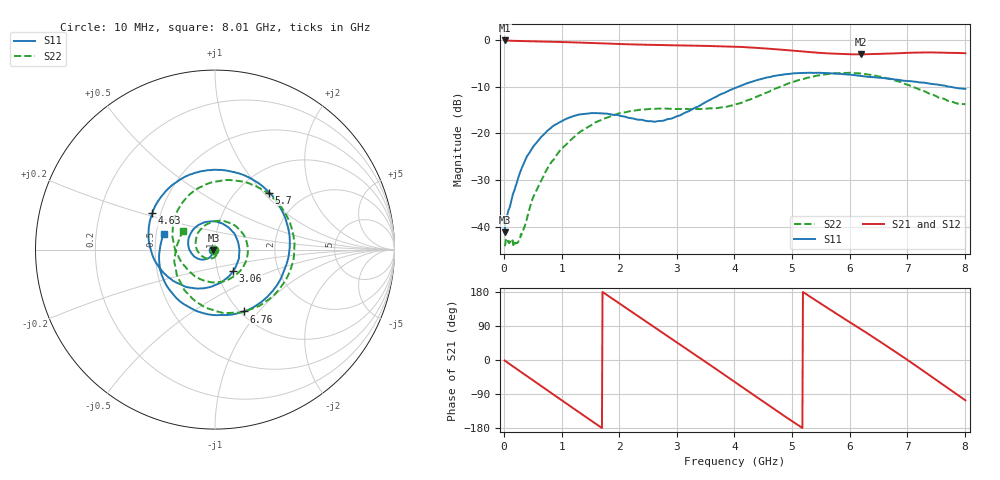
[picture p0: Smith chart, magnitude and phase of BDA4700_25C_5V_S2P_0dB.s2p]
!Agilent Technologies,E5071B,MY42404982,A.09.10
!Date: Mon Oct 20 13:25:59 2025
!Data & Calibration Information:
!Freq	S11:SOLT2(ON)	S21:SOLT2(ON)	S12:SOLT2(ON)	S22:SOLT2(ON)
# Hz S RI R 50
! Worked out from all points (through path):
!   801 points, 10 MHz to 8.01 GHz, reference 50 ohm
!   highest |S21| = -0.12 dB at 10 MHz (marker M1); lowest = -3.1 dB at 6.19 GHz (marker M2)
!   group delay of S21, straight-line fit = 285 ps
!   lowest |S11| = -41.1 dB at 10 MHz (marker M3), VSWR 1.02, Z = 49.2 - j0.259 ohm
!   |S11| at or under -10 dB: start of sweep to 4.065 GHz; 7.731 GHz to end of sweep
!   |S22| runs from -44.1 to -7.0 dB; largest |S21 - S12| = 0.0073
!   S11 on the Smith chart (normalised r, x): 10 MHz: 0.98, -0.01; 3.06 GHz: 1.18, -0.29; 4.63 GHz: 0.45, +0.22; 5.7 GHz: 1.37, +1.08; 6.76 GHz: 1.04, -0.84; 8.01 GHz: 0.55, +0.10
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1e7  -0.00836 -0.00263  0.9858 -0.0211  0.9859 -0.0221  -0.00624 -0.00044
2.6e8  -0.0186 -0.0303  0.859 -0.4568  0.8594 -0.457  0.00486 0.00556
7.2e8  -0.0874 -0.053  0.2215 -0.9322  0.2211 -0.9327  0.00204 -0.0389
1.02e9  -0.1369 -0.0116  -0.2964 -0.9004  -0.297 -0.9006  -0.0519 -0.0479
1.35e9  -0.144 0.0705  -0.7449 -0.5637  -0.7455 -0.5638  -0.1056 0.0151
1.92e9  -0.0155 0.1577  -0.8401 0.3442  -0.8409 0.3448  0.000695 0.1584
2.32e9  0.0934 0.1049  -0.3984 0.7978  -0.3985 0.7981  0.1469 0.1003
2.68e9  0.1358 0.00145  0.1593 0.8677  0.1596 0.8675  0.1779 -0.0486
3.06e9  0.0992 -0.1214  0.6655 0.5653  0.6626 0.5681  0.077 -0.1658
3.52e9  -0.0496 -0.2131  0.8552 -0.1075  0.8557 -0.109  -0.0892 -0.161
4.01e9  -0.2683 -0.1466  0.4427 -0.7199  0.4438 -0.7195  -0.1962 -0.0534
4.32e9  -0.3591 0.00465  -0.0123 -0.8256  -0.0129 -0.828  -0.232 0.0471
4.63e9  -0.3492 0.2019  -0.4405 -0.6699  -0.4398 -0.6707  -0.2232 0.1801
4.99e9  -0.1903 0.3929  -0.7229 -0.259  -0.7246 -0.26  -0.1035 0.3366
5.35e9  0.0677 0.4396  -0.7071 0.2095  -0.7083 0.2077  0.1265 0.3827
5.7e9  0.3022 0.3177  -0.4514 0.5529  -0.4508 0.5542  0.3483 0.2639
6.19e9  0.4119 -0.0265  0.0996 0.6931  0.1053 0.6948  0.4265 -0.0925
6.68e9  0.214 -0.3211  0.5975 0.3909  0.5995 0.3904  0.1805 -0.3385
6.76e9  0.1605 -0.3445  0.6487 0.3048  0.651 0.3025  0.1273 -0.3514
7.29e9  -0.1906 -0.2919  0.6359 -0.3657  0.6359 -0.3672  -0.167 -0.2298
7.65e9  -0.3073 -0.1049  0.2733 -0.6762  0.2711 -0.6773  -0.2262 -0.0553
8.01e9  -0.2868 0.0865  -0.203 -0.6898  -0.2017 -0.6912  -0.179 0.101
